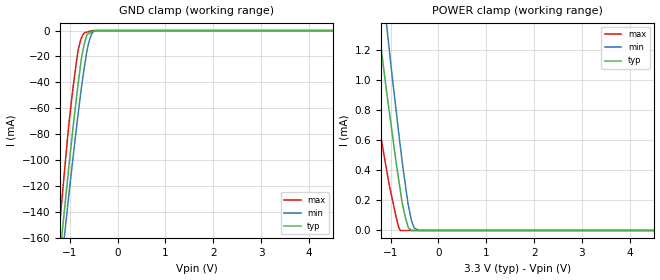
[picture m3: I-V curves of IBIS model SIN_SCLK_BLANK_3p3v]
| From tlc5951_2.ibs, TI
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|   sin_sclk_blank_3p3v Model
[Model]   SIN_SCLK_BLANK_3p3v
Model_type   Input
Vinl = 0.99
Vinh = 2.31
|   typ   min   max
|   (nom PVT)   (Fast PVT)   (slow PVT)
|Average
C_comp   1.245e-12   1.244e-12   1.262e-12
| Where nom  PVT is Nominal Process,  3.3V,  65C
|   Fast PVT is Strong Process,   3.6V,  -40C
|   Slow PVT is Weak Process,   3V,  125C
[Model Spec]
Vinl   0.99   0.9   1.08
Vinh   2.31   2.1   2.52
[Voltage Range]   3.3   3   3.6
|Ambient Temperature   25   85   -40
|Junction Temperature
[Temperature Range]   65   125   -40
[Power Clamp Reference]   3.3   3   3.6
[GND Clamp Reference]   0   0   0
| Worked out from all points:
|   GND clamp passes 1 mA (typ) near -0.54 V on its own axis
|   POWER clamp passes 1 mA (typ) near -1.11 V on its own axis
[GND Clamp]
|   Voltage   I(typ)   I(min)   I(max)
-3.3V     -1.048A    -1.001A    -1.1A
-1.267V   -197.3mA   -214.1mA   -174.4mA
-1.169V   -160.1mA   -179mA     -132.8mA
-1.139V   -148.7mA   -168.5mA   -120.5mA
-1.064V   -121.9mA   -142.8mA   -90.39mA
-931.2mV  -75.18mA   -98.1mA    -44.13mA
-823.2mV  -41.07mA   -64.13mA   -15.08mA
-759mV    -22.38mA   -44.99mA   -6.052mA
-686.4mV  -9.061mA   -26.39mA   -1.631mA
-555mV    -1.324mA   -3.66mA    -276.5uA
-411mV    0A         0A         0A
6.6V      0A         0A         0A
[POWER Clamp]
|   Voltage   I(typ)   I(min)   I(max)
-3.3V     6.588mA    5.352mA    5.817mA
-1.614V   2.338mA    2.995mA    1.43mA
-1.548V   2.148mA    2.791mA    1.294mA
-1.302V   1.483mA    2.026mA    810.1uA
-1.086V   928uA      1.371mA    406.4uA
-884.4mV  451.9uA    797.3uA    90.4uA
-798mV    268.4uA    561.2uA    0A
-689.7mV  83.97uA    299.6uA    0A
-627mV    16.22uA    163.5uA    0A
-561mV    0A         62.72uA    0A
-408mV    0A         0A         0A
6.6V      0A         0A         0A
